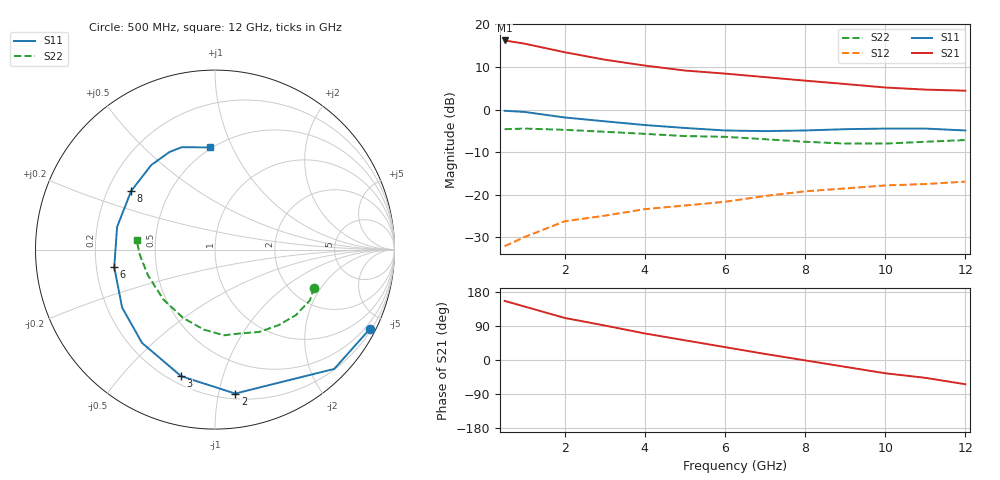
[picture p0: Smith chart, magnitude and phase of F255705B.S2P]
!ATF-25570
!S-PARAMETERS at Vds=5V  Id=50mA.  LAST UPDATED 07-22-92
# ghz s ma r 50
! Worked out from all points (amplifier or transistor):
!   13 points, 500 MHz to 12 GHz, reference 50 ohm
!   highest |S21| = 16.2 dB at 500 MHz (marker M1)
!   |S21| within 3 dB of that: start of sweep to 2.134 GHz
!   unconditionally stable (mu >= 1): 4.741 GHz to end of sweep
!   at 2 GHz: K = 0.55, MSG = 19.8 dB, |S12| = -26.2 dB
!   at 6 GHz: K = 1.09, MAG = 13.2 dB, |S12| = -21.6 dB
!   at 12 GHz: K = 1.02, MAG = 9.7 dB, |S12| = -16.9 dB
!   S11 on the Smith chart (normalised r, x): 500 MHz: 0.28, -4.15; 2 GHz: 0.24, -1.12; 3 GHz: 0.24, -0.74; 6 GHz: 0.28, -0.08; 8 GHz: 0.30, +0.29; 12 GHz: 0.49, +0.82
0.5  0.97 -27.0  6.49 156.0  0.025 63.0  0.59 -21.0
1  0.94 -45.0  5.95 141.0  0.032 57.0  0.6 -28.0
2  0.81 -82.0  4.72 111.0  0.049 45.0  0.58 -39.0
3  0.73 -105.0  3.86 91.0  0.057 41.0  0.55 -50.0
4  0.66 -128.0  3.29 70.0  0.068 37.0  0.52 -62.0
5  0.61 -148.0  2.88 52.0  0.075 32.0  0.49 -72.0
6  0.57 -170.0  2.65 34.0  0.083 30.0  0.48 -84.0
7  0.56 167.0  2.41 16.0  0.097 28.0  0.45 -98.0
8  0.57 145.0  2.19 -1.0  0.11 18.0  0.42 -115.0
9  0.59 127.0  2 -18.0  0.119 12.0  0.4 -136.0
10  0.6 115.0  1.82 -35.0  0.129 4.0  0.4 -159.0
11  0.6 108.0  1.72 -47.0  0.134 1.0  0.42 -176.0
12  0.57 93.0  1.67 -64.0  0.143 -10.0  0.44 173.0
